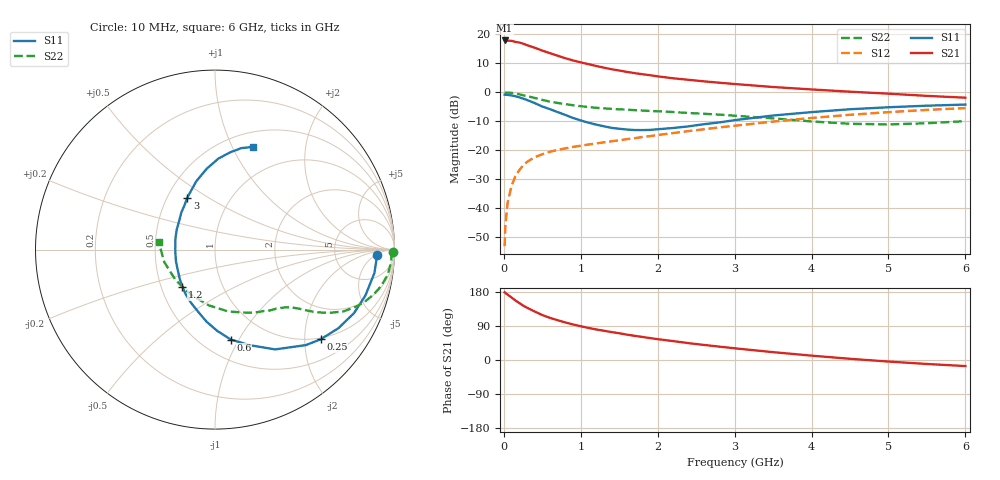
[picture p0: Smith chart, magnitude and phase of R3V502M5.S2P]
! SIEMENS Small Signal Semiconductors
! BFR181
! Si NPN RF Bipolar Junction Transistor in SOT23
! VCE = 0.5 V  IC = 2.5 mA
! Common Emitter S-Parameters:  May  1996
# GHz  S  MA  R  50
!  f  S11  S21  S12  S22
! GHz  MAG  ANG  MAG  ANG  MAG  ANG  MAG  ANG
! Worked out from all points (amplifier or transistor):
!   36 points, 10 MHz to 6 GHz, reference 50 ohm
!   highest |S21| = 17.8 dB at 10 MHz (marker M1)
!   |S21| within 3 dB of that: start of sweep to 449.9 MHz
!   unconditionally stable (mu >= 1): 1.194 GHz to 4.117 GHz
!   at 250 MHz: K = 0.30, MSG = 21.0 dB, |S12| = -25.3 dB
!   at 1.4 GHz: K = 1.08, MAG = 10.8 dB, |S12| = -17.0 dB
!   at 6 GHz: K = 0.96, MSG = 1.8 dB, |S12| = -5.5 dB
!   S11 on the Smith chart (normalised r, x): 10 MHz: 18, -6; 250 MHz: 0.96, -2.39; 600 MHz: 0.68, -0.93; 1.2 GHz: 0.64, -0.29; 3 GHz: 0.63, +0.41; 6 GHz: 0.66, +1.21
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0.01  0.9037 -1.8  7.805 178.7  0.0022 89.5  0.9898 -0.8
0.02  0.9018 -3.3  7.683 176.9  0.005 85.9  0.9841 -1.8
0.05  0.8976 -8.4  7.75 172.4  0.0126 84.2  0.9839 -4.2
0.1  0.8763 -16.9  7.684 165.0  0.0241 80.1  0.9717 -8.4
0.15  0.8513 -24.6  7.367 157.1  0.0354 75.4  0.948 -12.3
0.2  0.8151 -32.5  7.2 150.4  0.045 71.4  0.9196 -15.7
0.25  0.7725 -40.3  6.882 143.7  0.0543 67.5  0.8866 -18.9
0.3  0.7346 -46.4  6.48 138.0  0.0624 64.7  0.8548 -21.5
0.4  0.6494 -58.9  5.856 128.1  0.0754 59.4  0.7959 -25.6
0.5  0.5655 -70.2  5.212 118.5  0.0848 55.6  0.7351 -28.6
0.6  0.5089 -80.0  4.7 111.2  0.0938 53.4  0.6867 -30.7
0.8  0.4042 -96.7  3.85 99.1  0.1073 50.7  0.6206 -33.3
0.9  0.3587 -105.2  3.527 93.7  0.1137 50.1  0.5953 -34.2
1.1  0.2974 -123.4  3.041 84.7  0.1248 49.7  0.5539 -36.0
1.2  0.2753 -131.3  2.833 80.6  0.1304 49.7  0.5379 -36.9
1.6  0.2268 -163.7  2.236 66.9  0.1546 50.3  0.4985 -40.6
2.2  0.2408 152.3  1.736 49.9  0.1969 50.4  0.4544 -48.4
3  0.3287 118.0  1.383 30.9  0.2634 47.7  0.3927 -63.4
3.5  0.3954 105.2  1.227 20.7  0.3108 44.2  0.3533 -77.7
4.5  0.5073 87.9  1.019 3.2  0.4071 34.0  0.2847 -118.6
5.5  0.5843 75.4  0.863 -10.5  0.4943 21.7  0.2908 -166.0
6  0.6112 69.5  0.803 -16.0  0.531 14.8  0.3163 172.5
